(* Logix 5000 AddOnInstructionDefinition export AMCI_SD4840E2_Home_CCW; software revision 20.03 *)

ADD_ON_INSTRUCTION AMCI_SD4840E2_Home_CCW   (* revision 1.0, vendor AMCI, ExecuteEnableInFalse *)
VAR_INPUT
   Axis_Status_Bits : INT; {required}
   Type_0_for_standard_1_for_indexed : BOOL;
   Programmed_Speed : DINT; {required}
   Acceleration : INT; {required}
   Deceleration : INT; {required}
   Jerk : INT;
END_VAR
VAR_IN_OUT
   AMCI_SD4840E2_output_data : _000A:SD4840E2_4342D302:O:0; {required}
END_VAR
VAR_OUTPUT
   EN : BOOL; {access Read Only, visible}
   ER : BOOL; {access Read Only, visible}
END_VAR
VAR
   Upper_Result_X_1000 : DINT;
   command_data_block : INT[10];
        [0]   // Command Bits MSW
        [1]   // Command Bits LSW
        [2]   // Upper Target Position
        [3]   // Lower Target Position
        [4]   // Upper Programmed Speed
        [5]   // Lower Programmed Speed
END_VAR

ROUTINE EnableInFalse   (* ladder *)
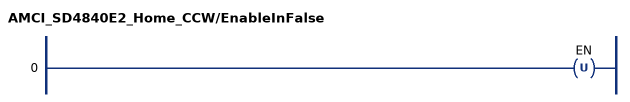
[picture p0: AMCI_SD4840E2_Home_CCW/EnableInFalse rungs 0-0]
   0: OTU(EN);
END_ROUTINE

ROUTINE Logic   (* ladder *)
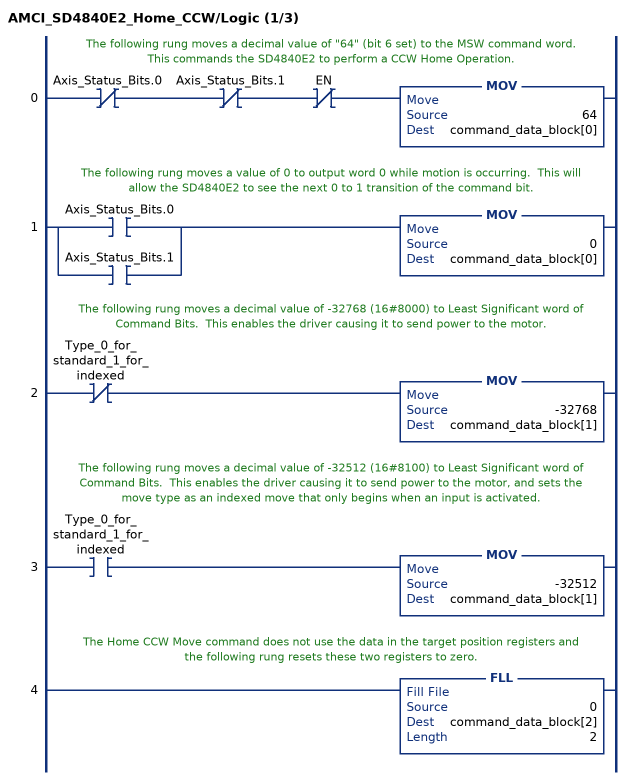
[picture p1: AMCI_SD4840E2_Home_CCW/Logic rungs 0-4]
   // The following rung moves a decimal value of "64" (bit 6 set) to the MSW command word.  This commands the SD4840E2 to perform a CCW Home Operation.
   0: XIO(Axis_Status_Bits.0)XIO(Axis_Status_Bits.1)XIO(EN)MOV(64,command_data_block[0]);
   // The following rung moves a value of 0 to output word 0 while motion is occurring.  This will allow the SD4840E2 to see the next 0 to 1 transition of the command bit.
   1: [XIC(Axis_Status_Bits.0) ,XIC(Axis_Status_Bits.1) ]MOV(0,command_data_block[0]);
   // The following rung moves a decimal value of -32768 (16#8000) to Least Significant word of Command Bits.  This enables the driver causing it to send power to the motor.
   2: XIO(Type_0_for_standard_1_for_indexed)MOV(-32768,command_data_block[1]);
   // The following rung moves a decimal value of -32512 (16#8100) to Least Significant word of Command Bits.  This enables the driver causing it to send power to the motor, and sets the move type as an indexed move that only begins when an input is activated.
   3: XIC(Type_0_for_standard_1_for_indexed)MOV(-32512,command_data_block[1]);
   // The Home CCW Move command does not use the data in the target position registers and the following rung resets these two registers to zero.
   4: FLL(0,command_data_block[2],2);
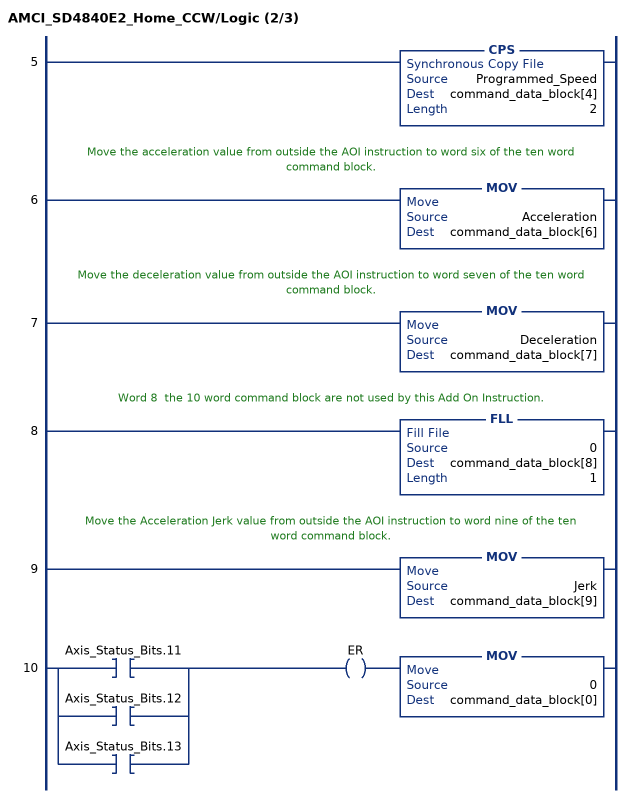
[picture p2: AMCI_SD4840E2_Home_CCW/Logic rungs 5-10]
   5: CPS(Programmed_Speed,command_data_block[4],2);
   // Move the acceleration value from outside the AOI instruction to word six of the ten word command block.
   6: MOV(Acceleration,command_data_block[6]);
   // Move the deceleration value from outside the AOI instruction to word seven of the ten word command block.
   7: MOV(Deceleration,command_data_block[7]);
   // Word 8  the 10 word command block are not used by this Add On Instruction.
   8: FLL(0,command_data_block[8],1);
   // Move the Acceleration Jerk value from outside the AOI instruction to word nine of the ten word command block.
   9: MOV(Jerk,command_data_block[9]);
   10: [XIC(Axis_Status_Bits.11) ,XIC(Axis_Status_Bits.12) ,XIC(Axis_Status_Bits.13) ]OTE(ER)MOV(0,command_data_block[0]);
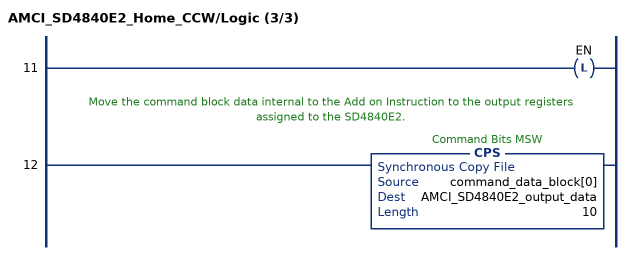
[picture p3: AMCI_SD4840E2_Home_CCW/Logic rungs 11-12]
   11: OTL(EN);
   // Move the command block data internal to the Add on Instruction to the output registers assigned to the SD4840E2.
   12: CPS(command_data_block[0],AMCI_SD4840E2_output_data,10);
END_ROUTINE
END_ADD_ON_INSTRUCTION
